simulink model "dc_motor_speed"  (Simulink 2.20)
settings: Solver=FixedStepDiscrete  StartTime=0.0  StopTime=5.0  FixedStep=0.12  RelTol=1e-3  AbsTol=1e-6

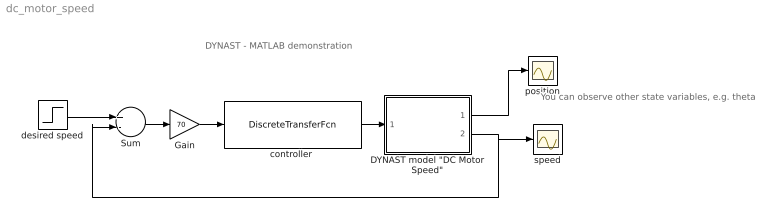
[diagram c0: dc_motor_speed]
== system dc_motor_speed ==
  note: DYNAST - MATLAB demonstration
  note: You can observe other state variables, e.g. theta
  "DYNAST model \"DC Motor Speed\"" : Subsystem
  Gain : Gain  Gain=70
  Sum : Sum  Inputs=+-
  "controller " : DiscreteTransferFcn  Numerator="[1.0000   -1.1100    0.2823]"  Denominator="[1.6000   -0.6000   -1.0000]"  SampleTime=0.12
  desired speed : Step  Time=0  Before=0  After=1
  position : Scope
  speed : Scope
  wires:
  Sum/1 -> Gain/1
  Gain/1 -> "controller "/1
  "controller "/1 -> "DYNAST model \"DC Motor Speed\""/1(V)
  "DYNAST model \"DC Motor Speed\""/2(thetadot) -> speed/1, Sum/2
  "DYNAST model \"DC Motor Speed\""/1(theta) -> position/1
  desired speed/1 -> Sum/1

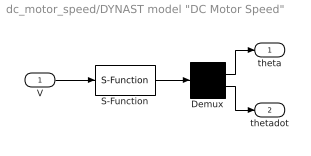
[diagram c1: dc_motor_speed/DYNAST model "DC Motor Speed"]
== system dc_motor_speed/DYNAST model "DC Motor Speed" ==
  V : Inport  Port=1  PortWidth=-1  SampleTime=-1
  Demux : Demux  Outputs=2
  S-Function : S-Function  FunctionName=dynPlantL  Parameters='%DYNAST%\examples\control\DCMotorSpeed.prb',0.12  PortCounts=[]  SFunctionModules=''
  theta : Outport  Port=1
  thetadot : Outport  Port=2
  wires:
  V/1 -> S-Function/1
  S-Function/1 -> Demux/1
  Demux/1 -> theta/1
  Demux/2 -> thetadot/1
